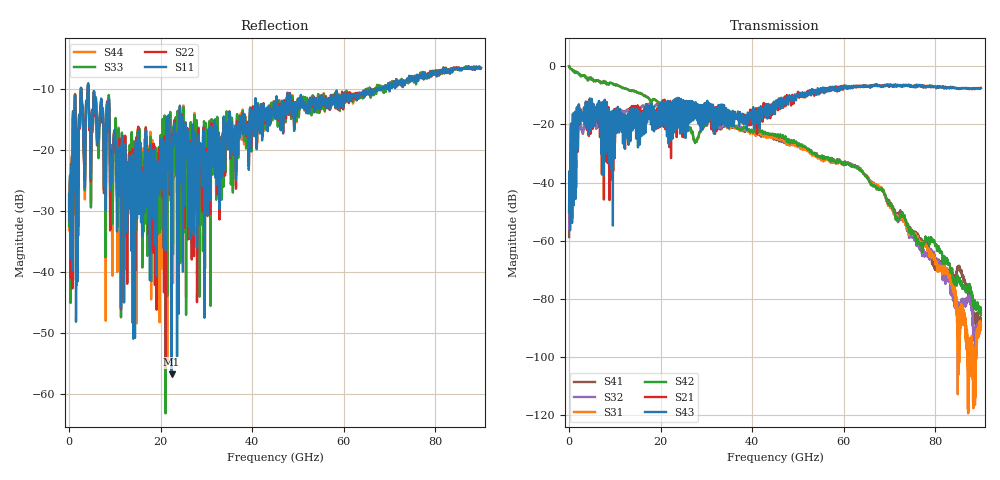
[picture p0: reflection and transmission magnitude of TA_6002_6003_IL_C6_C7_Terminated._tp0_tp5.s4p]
!Touchstone File created by Channel Assembly Engine (Version 2.0.0_Beta1)
!Current time:  2022 6/29 11:33:40
!Port 1 -> Port 3 : Port 3 Device 1 (Port3) -> Port 4 Device 6 (Port4)
!Port 2 -> Port 4 : Port 4 Device 1 (Port4) -> Port 3 Device 6 (Port3)
!Port 3 -> Port 1 : Port 4 Device 6 (Port4) -> Port 3 Device 1 (Port3)
!Port 4 -> Port 2 : Port 3 Device 6 (Port3) -> Port 4 Device 1 (Port4)
# Hz S RI R 50
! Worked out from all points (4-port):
!   9000 points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, 10 MHz to 90 GHz, reference 50 ohm
!   strongest paths, dB at 10 MHz, 22.51 GHz, 45.01 GHz, 67.51 GHz, 90 GHz:
!     S43: -50.0, -16.0, -15.9, -6.8, -7.5
!     S21: -50.1, -12.8, -12.7, -6.7, -7.5
!     S42: 0.0, -16.2, -23.4, -41.8, -84.8
!     S31: 0.0, -16.4, -24.2, -40.9, -89.7
!     S32: -55.9, -13.6, -24.1, -41.4, -89.8
!     S41: -58.7, -13.4, -24.6, -41.1, -88.6
!   lowest |S11| = -56.7 dB at 22.4 GHz (marker M1), VSWR 1.00, Z = 50.1 + j0.136 ohm
!   |S11| at or under -10 dB: start of sweep to 2.574 GHz; 2.65 GHz to 4.062 GHz (1.412 GHz wide, 42.1 % of centre); 4.242 GHz to 67.1 GHz (62.86 GHz wide, 176 % of centre)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
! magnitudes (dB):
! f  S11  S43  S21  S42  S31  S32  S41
! 10 MHz  -27.2  -50.0  -50.1  0.0  0.0  -55.9  -58.7
! 770 MHz  -21.4  -19.6  -19.7  -1.4  -1.4  -24.2  -24.1
! 2.35 GHz  -16.2  -19.7  -19.8  -2.8  -2.8  -20.1  -20.1
! 12.69 GHz  -31.9  -18.9  -22.8  -7.9  -7.9  -15.1  -15.0
! 22.4 GHz  -56.7  -12.7  -14.3  -16.2  -16.4  -13.6  -13.4
! 63.35 GHz  -11.4  -6.9  -6.8  -35.4  -35.2  -35.3  -35.0
! 90 GHz  -6.5  -7.5  -7.5  -84.8  -89.7  -89.8  -88.6
